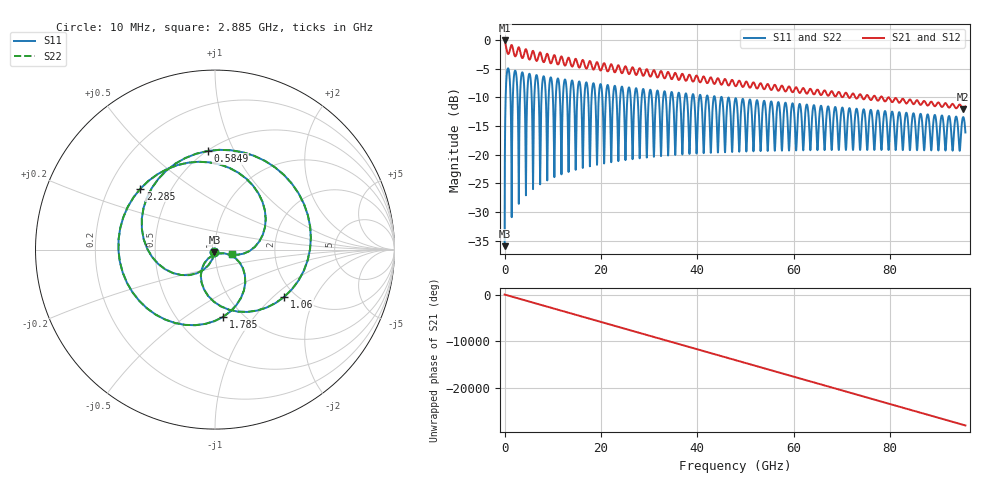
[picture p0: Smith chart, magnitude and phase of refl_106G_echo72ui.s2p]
! Created with skrf 1.10.0 (http://scikit-rf.org).
# GHz S RI R 50.0
!freq ReS11 ImS11 ReS21 ImS21 ReS12 ImS12 ReS22 ImS22
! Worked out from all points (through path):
!   3826 points, 10 MHz to 95.62 GHz, reference 50 ohm
!   highest |S21| = -0.07 dB at 10 MHz (marker M1); lowest = -12.0 dB at 95.2 GHz (marker M2)
!   group delay of S21, straight-line fit = 816 ps
!   lowest |S11| = -35.9 dB at 10 MHz (marker M3), VSWR 1.03, Z = 49.7 - j1.56 ohm
!   |S11| at or under -10 dB: 42.21 GHz to 43.4 GHz (1.195 GHz wide, 2.79 % of centre); 43.66 GHz to 44.92 GHz (1.264 GHz wide, 2.85 % of centre); 45.09 GHz to end of sweep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
!   |S22| runs from -35.9 to -4.9 dB; largest |S21 - S12| = 4e-16
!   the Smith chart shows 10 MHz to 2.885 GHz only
!   S11 on the Smith chart (normalised r, x): 10 MHz: 0.99, -0.03; 584.9 MHz: 0.50, +0.79; 1.06 GHz: 1.75, -1.18; 1.785 GHz: 0.81, -0.71; 2.285 GHz: 0.34, +0.32; 2.885 GHz: 1.21, -0.06
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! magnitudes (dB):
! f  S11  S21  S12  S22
! 10 MHz  -35.9  -0.1  -0.1  -35.9
! 584.9 MHz  -5.2  -2.2  -2.2  -5.2
! 1.06 GHz  -6.6  -1.9  -1.9  -6.6
! 1.785 GHz  -8.5  -1.7  -1.7  -8.5
! 2.285 GHz  -5.4  -2.8  -2.8  -5.4
! 2.885 GHz  -20.2  -1.3  -1.3  -20.2
! 3.685 GHz  -5.6  -3.1  -3.1  -5.6
! 4.41 GHz  -26.2  -1.6  -1.6  -26.2
! 5.159 GHz  -5.9  -3.4  -3.4  -5.9
! 5.884 GHz  -25.2  -1.9  -1.9  -25.2
! 6.634 GHz  -6.1  -3.6  -3.6  -6.1
! 7.359 GHz  -24.5  -2.1  -2.1  -24.5
! 8.109 GHz  -6.3  -3.8  -3.8  -6.3
! 8.834 GHz  -23.8  -2.4  -2.4  -23.8
! 9.584 GHz  -6.5  -4.1  -4.1  -6.5
! 15.96 GHz  -11.3  -3.9  -3.9  -11.3
! 31.88 GHz  -9.1  -6.4  -6.4  -9.1
! 47.83 GHz  -10.4  -8.0  -8.0  -10.4
! 63.75 GHz  -14.3  -8.9  -8.9  -14.3
! 79.7 GHz  -19.2  -10.0  -10.0  -19.2
! 95.2 GHz  -13.4  -12.0  -12.0  -13.4
! 95.62 GHz  -16.1  -11.6  -11.6  -16.1
